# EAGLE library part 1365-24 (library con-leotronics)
DUAL ROW STRAIGHT HEADER 1364 SERIES. 1.27mm x 1.27mm. Without Fixing Post. SMT Source: http://www.leotronics.co.uk/Conexcon/Data%20Sheets/sec.%20A/1364ing.pdf
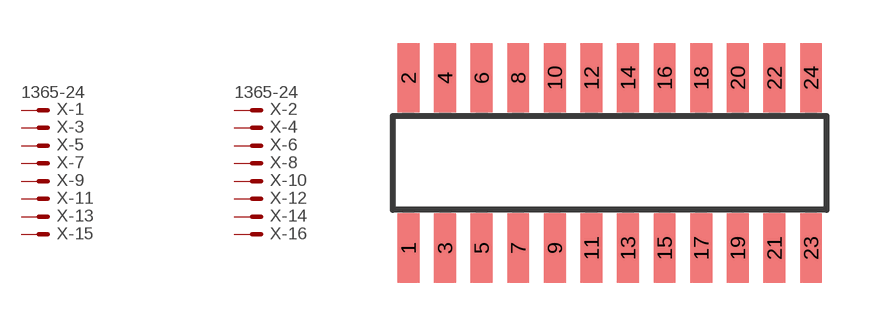
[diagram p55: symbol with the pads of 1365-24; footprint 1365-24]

Designator prefix X; gates -1=MVAL -2=MVAL -3=M -4=M -5=M -6=M -7=M -8=M -9=M -10=M -11=M -12=M -13=M -14=M -15=M -16=M -17=M -18=M -19=M -20=M -21=M -22=M -23=M -24=M

## 1365-24 (OC_FARNELL: unknown; OC_NEWARK: unknown)  [1365-24]
1  -1:S  pas
2  -2:S  pas
3  -3:S  pas
4  -4:S  pas
5  -5:S  pas
6  -6:S  pas
7  -7:S  pas
8  -8:S  pas
9  -9:S  pas
10  -10:S  pas
11  -11:S  pas
12  -12:S  pas
13  -13:S  pas
14  -14:S  pas
15  -15:S  pas
16  -16:S  pas
17  -17:S  pas
18  -18:S  pas
19  -19:S  pas
20  -20:S  pas
21  -21:S  pas
22  -22:S  pas
23  -23:S  pas
24  -24:S  pas

## Footprint 1365-24 (pad centres in mm)
DUAL ROW STRAIGHT HEADER 1364 SERIES. 1.27mm x 1.27mm. Without Fixing Post. SMT Source: http://www.leotronics.co.uk/Conexcon/Data%20Sheets/sec.%20A/1364ing.pdf
smd 0.76 x 2.4: 1 -6.985,-2.95; 2 -6.985,2.95; 3 -5.715,-2.95; 4 -5.715,2.95; 5 -4.445,-2.95; 6 -4.445,2.95; 7 -3.175,-2.95; 8 -3.175,2.95; 9 -1.905,-2.95; 10 -1.905,2.95; 11 -0.635,-2.95; 12 -0.635,2.95; 13 0.635,-2.95; 14 0.635,2.95; 15 1.905,-2.95; 16 1.905,2.95; 17 3.175,-2.95; 18 3.175,2.95; 19 4.445,-2.95; 20 4.445,2.95; 21 5.715,-2.95; 22 5.715,2.95; 23 6.985,-2.95; 24 6.985,2.95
